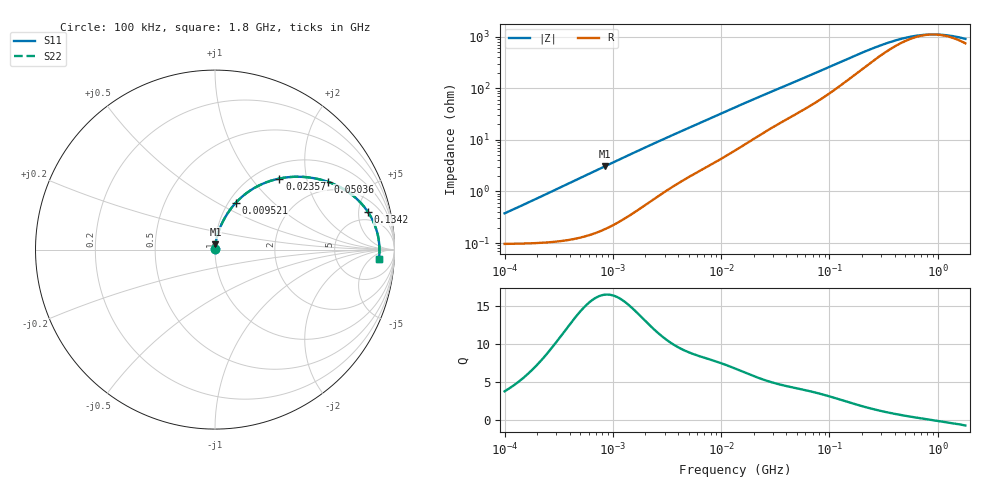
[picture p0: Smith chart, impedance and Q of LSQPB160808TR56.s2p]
! LSQPB160808TR56  S-PARAMETER MODEL  ( General Type )
! Model Generated by TAIYO YUDEN Corporation (http://www.ty-top.com)
! Version 4.0
! TAIYO YUDEN Control No. 100810NF18SB-HKC
! Copyright(c) 2007 TAIYO YUDEN CO.,LTD. All Rights Reserved.
! Product Description (link to TY-COMPAS)
! https://ds.yuden.co.jp/TYCOMPAS/or/detail?pn=LSQPB160808TR56M&u=M
! Products Name : Inductors
! Characteristics :
!  Inductance : 0.56 uH , SRF(min) : 170 MHz , DC Resistance(max) : 0.1235 Ohm
!  Rated Current : Saturation :1150 mA , Temp Rise : 760 mA (40 degC)
!  Case Size : 1.6 x 0.8 / 0.063 x 0.031 [mm/inch] , Thickness : 0.8 / 0.031 [mm/inch]
!  (Conditions: Temperature = 25 degC , DC Bias Current/Voltage = 0A / 0V)
! External Node Assignments :
!  1  o---GGG---o  2
! GND o---------o GND
! Frequency Range : 0.1MHz  -  1800MHz  [ 402 STEP ]
# MHz S RI R 50
! Freq[MHz].  S11 Real  S11 Imag  S21 Real  S21 Imag  S12 Real  S12 Imag  S22 Real  S22 Imag
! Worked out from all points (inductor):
!   401 points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, 100 kHz to 1.8 GHz, reference 50 ohm
!   read as one part in series: L = 580 nH near 105 kHz
!   highest Q = 16.5 at 842.4 kHz (marker M1), where L = 577 nH
!   self-resonance near 900.8 MHz
!   S11 on the Smith chart (normalised r, x): 100 kHz: 1.00, +0.01; 9.521 MHz: 1.08, +0.61; 23.57 MHz: 1.26, +1.40; 50.36 MHz: 1.65, +2.70; 134.2 MHz: 3.47, +6.33; 1.8 GHz: 16, -10
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0.1  0.000975 0.00364  0.999 -0.00364  0.999 -0.00364  0.000975 0.00364
0.151652  0.00101 0.00551  0.999 -0.00551  0.999 -0.00551  0.00101 0.00551
0.516129  0.00165 0.0187  0.9984 -0.0187  0.9984 -0.0187  0.00165 0.0187
0.842407  0.00278 0.0304  0.9972 -0.0304  0.9972 -0.0304  0.00278 0.0304
1.55409  0.0069 0.0552  0.9931 -0.0552  0.9931 -0.0552  0.0069 0.0552
2.66389  0.0167 0.0913  0.9833 -0.0913  0.9833 -0.0913  0.0167 0.0913
5.554714  0.0523 0.1722  0.9477 -0.1722  0.9477 -0.1722  0.0523 0.1722
9.52142  0.1152 0.26  0.8848 -0.26  0.8848 -0.26  0.1152 0.26
13.41641  0.1856 0.3219  0.8144 -0.3219  0.8144 -0.3219  0.1856 0.3219
17.56533  0.2607 0.3646  0.7393 -0.3646  0.7393 -0.3646  0.2607 0.3646
23.56755  0.359 0.396  0.641 -0.396  0.641 -0.396  0.359 0.396
34.03197  0.4927 0.4049  0.5073 -0.4049  0.5073 -0.4049  0.4927 0.4049
50.36143  0.6299 0.3774  0.3701 -0.3774  0.3701 -0.3774  0.6299 0.3774
69.24595  0.725 0.332  0.275 -0.332  0.275 -0.332  0.725 0.332
95.21179  0.7982 0.2746  0.2018 -0.2746  0.2018 -0.2746  0.7982 0.2746
134.1607  0.8513 0.2109  0.1487 -0.2109  0.1487 -0.2109  0.8513 0.2109
208.5031  0.889 0.1395  0.111 -0.1395  0.111 -0.1395  0.889 0.1395
357.3983  0.9085 0.0747  0.0915 -0.0747  0.0915 -0.0747  0.9085 0.0747
542.0029  0.9142 0.0376  0.0858 -0.0376  0.0858 -0.0376  0.9142 0.0376
802.0705  0.9162 0.00828  0.0838 -0.00828  0.0838 -0.00828  0.9162 0.00828
1186.925  0.9161 -0.0199  0.0839 0.0199  0.0839 0.0199  0.9161 -0.0199
1800  0.9135 -0.0532  0.0865 0.0532  0.0865 0.0532  0.9135 -0.0532
